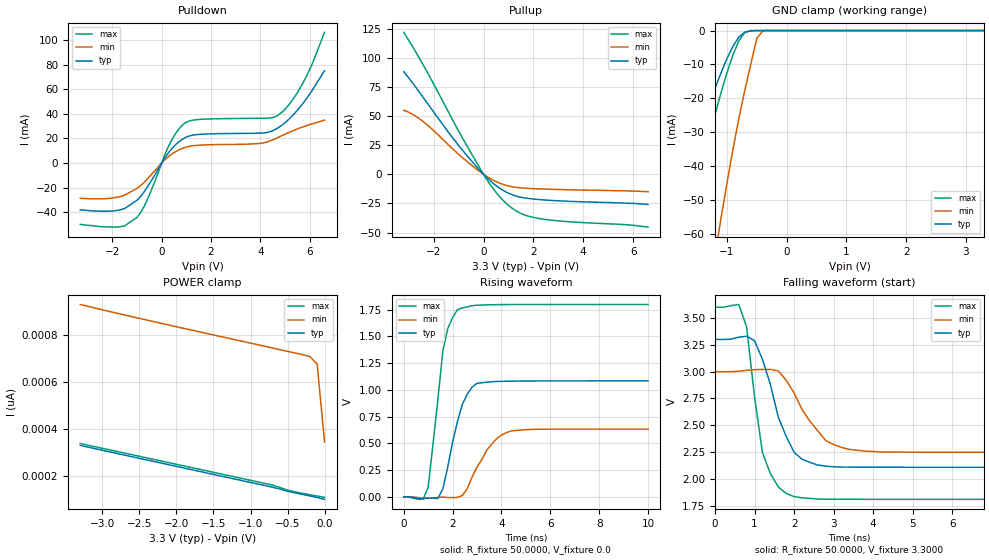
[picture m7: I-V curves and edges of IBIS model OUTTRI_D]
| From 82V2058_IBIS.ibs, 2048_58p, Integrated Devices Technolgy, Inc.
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|   Model OUTTRI_D
[Model]   OUTTRI_D
Model_type   3-state
Polarity   Non-Inverting
Enable   Active-Low
Vmeas =   1.65V
C_comp   2.6600pF   2.5500pF   2.7500pF
[Temperature Range]   25.0000   85.0000   -40.0000
[Voltage Range]   3.3000V   3.0000V   3.6000V
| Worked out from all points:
|   slope of the pulldown table from 0 to 0.495 V, typ, clamps not added: 36.6 ohm
|   slope of the pullup table from 0 to 0.495 V, typ, clamps not added: 51.8 ohm
|   GND clamp passes 1 mA (typ) near -0.74 V on its own axis
|   rising waveform, R_fixture 50.0000, V_fixture 0.0: 20-80 % time 663ps typ, 961ps min, 539ps max; typ from 0 V to 1.08 V
|   falling waveform, R_fixture 50.0000, V_fixture 3.3000: 20-80 % time 623ps typ, 790ps min, 426ps max; typ from 3.3 V to 2.11 V
[Pulldown]
|Voltage   I(typ)   I(min)   I(max)
-3.3V     -38mA      -28.6mA    -49.8mA
-1.7V     -38.12mA   -27.3mA    -51.77mA
-1V       -30.16mA   -20.54mA   -44.11mA
-600mV    -20.06mA   -13.26mA   -30.47mA
400mV     11.46mA    7.126mA    18.48mA
700mV     17.32mA    10.72mA    27.8mA
1V        21.1mA     13.02mA    33.19mA
4.2V      24.59mA    16.74mA    36.49mA
4.9V      31.19mA    22.56mA    41.78mA
5.7V      47.8mA     29.22mA    64.13mA
6.1V      59.04mA    31.92mA    80.46mA
6.6V      75.04mA    34.89mA    106.2mA
[Pullup]
|Voltage   I(typ)   I(min)   I(max)
-3.2V     88.08mA    54.91mA    121.9mA
-2.8V     77.12mA    50.95mA    108mA
-2.4V     65.44mA    44.93mA    93.18mA
-1V       24.75mA    17.16mA    37.07mA
0V        -6.24pA    -41.8pA    -5.2pA
300mV     -6.154mA   -3.996mA   -9.798mA
600mV     -11.19mA   -7.142mA   -18.04mA
1.1V      -17.14mA   -10.52mA   -28.36mA
1.6V      -20.15mA   -11.83mA   -34.51mA
2.4V      -21.99mA   -12.66mA   -38.54mA
5.7V      -24.77mA   -14.2mA    -43.26mA
6.6V      -25.9mA    -15mA      -45.4mA
[GND_clamp]
|Voltage   I(typ)   I(min)   I(max)
-3.3V     -132.9mA   -313.8mA   -170.5mA
-2V       -60.27mA   -158.7mA   -81.36mA
-1.9V     -54.57mA   -146.8mA   -74.16mA
-1.7V     -43.29mA   -123.2mA   -59.73mA
-1.2V     -17.04mA   -66.29mA   -24.77mA
-1.1V     -12.49mA   -55.5mA    -18.39mA
-900mV    -4.677mA   -35.12mA   -7.203mA
-800mV    -1.874mA   -25.89mA   -2.998mA
-700mV    -481.7uA   -17.58mA   -563.2uA
-500mV    -16.62uA   -2.324mA   -1.086uA
-400mV    -424.8nA   -91.35uA   -22.54nA
3.3V      102.4pA    717.1pA    94.7pA
[POWER_clamp]
|Voltage   I(typ)   I(min)   I(max)
-3.3V     331.5pA    929.8pA    339.6pA
-2.3V     262.9pA    856.6pA    271.6pA
-700mV    153.7pA    744.9pA    162.7pA
-500mV    137pA      730.9pA    141.3pA
-200mV    116.9pA    709.2pA    122pA
-100mV    110.2pA    677pA      116.5pA
0V        102.5pA    346.3pA    111.1pA
[Ramp]
| variable   typ   min   max
dV/dt_r   0.6504/0.6573n   0.3792/0.9370n   1.0782/0.4516n
dV/dt_f   0.7146/0.5786n   0.4506/0.7868n   1.0734/0.4000n
R_load =   50.0000
[Rising Waveform]
R_fixture=   50.0000
V_fixture=   0.0
V_fixture_min=  0.0
V_fixture_max=  0.0
|time   V(typ)   V(min)   V(max)
0s        0V         0V         0V
800ps     -18.7mV    -12.55mV   -18.53mV
1ns       -9.732mV   -14.69mV   88.98mV
1.6ns     74.9mV     -2.619mV   1.361V
1.8ns     275.6mV    -6.793mV   1.571V
2.2ns     704.4mV    -5.24mV    1.749V
2.8ns     1.025V     186.1mV    1.786V
3.4ns     1.071V     437.2mV    1.794V
4.2ns     1.08V      599.5mV    1.796V
10ns      1.084V     632mV      1.797V
[Falling Waveform]
R_fixture=   50.0000
V_fixture=   3.3000
V_fixture_min=  3.0000
V_fixture_max=  3.6000
|time   V(typ)   V(min)   V(max)
0s        3.3V       3V         3.6V
600ps     3.321V     3.004V     3.625V
800ps     3.33V      3.012V     3.418V
1ns       3.289V     3.019V     2.763V
1.2ns     3.114V     3.02V      2.247V
1.8ns     2.397V     2.921V     1.867V
2.2ns     2.184V     2.649V     1.825V
2.8ns     2.12V      2.358V     1.812V
3.4ns     2.111V     2.276V     1.812V
10ns      2.109V     2.249V     1.811V
